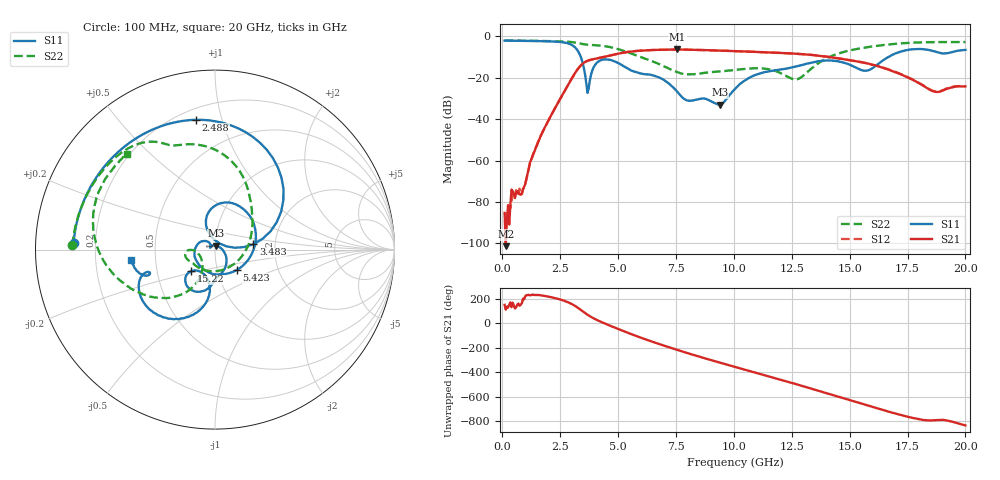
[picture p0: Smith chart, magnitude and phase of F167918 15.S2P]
!  2-Port S-parameters saved by WinCal
! VAR MeasName=S-Parameters (CALIBRATED_DATA) read from VNA (N5242A)
! VAR MeasDate=2016-11-22 10:25:31
! VAR NAME=F167918 15
! VAR FILENAME=F167918 15.S2P
! VAR DATE=2016-11-22 10:25:31
! VAR PHYS_PORTS=1,2
# Hz S DB R 50
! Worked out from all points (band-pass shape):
!   401 points, 100 MHz to 20 GHz, reference 50 ohm
!   highest |S21| = -6.37 dB at 7.562 GHz (marker M1); lowest = -101.4 dB at 149.8 MHz (marker M2)
!   |S21| within 3 dB of the highest: 4.617 GHz to 13.66 GHz (9.042 GHz wide, 98.9 % of centre)
!   lowest |S11| = -33.1 dB at 9.403 GHz (marker M3), VSWR 1.05, Z = 50.7 + j2.14 ohm
!   |S11| at or under -10 dB: 3.391 GHz to 16.67 GHz (13.28 GHz wide, 132 % of centre)
!   |S22| runs from -20.9 to -2.0 dB; largest |S21 - S12| = 0.0044
!   S11 on the Smith chart (normalised r, x): 100 MHz: 0.12, +0.02; 2.488 GHz: 0.27, +0.83; 3.483 GHz: 1.54, +0.10; 5.423 GHz: 1.24, -0.29; 15.22 GHz: 0.74, -0.19; 20 GHz: 0.36, -0.05
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1e8  -2.07 177.3  -85.33 148.6  -85.97 171.1  -2.00 178.3
1.4975e8  -2.07 176.0  -101.39 109.5  -85.49 150.5  -2.01 177.5
8.96e8  -2.18 156.0  -73.81 -160.8  -73.68 177.3  -2.12 165.5
1.44325e9  -2.28 140.1  -53.92 -131.0  -53.94 -129.4  -2.20 156.6
2.488e9  -2.72 98.3  -30.49 -166.7  -30.50 -167.3  -2.43 137.4
3.085e9  -4.78 52.6  -18.76 146.7  -18.78 146.5  -2.91 123.2
3.43325e9  -11.35 12.7  -13.60 101.9  -13.59 101.9  -3.66 115.7
3.483e9  -13.30 8.0  -13.12 95.0  -13.10 94.9  -3.76 115.0
3.682e9  -27.33 51.7  -11.84 68.4  -11.81 68.2  -4.06 112.3
4.279e9  -11.43 78.2  -10.24 9.0  -10.24 8.7  -4.55 99.3
5.42325e9  -15.60 -43.3  -7.56 -78.7  -7.55 -78.7  -7.74 65.5
6.7665e9  -19.84 163.3  -6.50 -169.8  -6.50 -170.0  -13.40 20.3
7.5625e9  -26.89 129.5  -6.37 141.6  -6.40 141.5  -17.35 -33.6
9.40325e9  -33.05 71.2  -6.90 38.2  -6.91 38.2  -16.93 -144.5
1.005e10  -25.37 -15.8  -7.13 3.7  -7.15 3.8  -16.27 -155.2
1.169175e10  -16.57 -82.2  -7.88 -82.9  -7.85 -82.8  -16.46 -178.4
1.268675e10  -14.55 -93.3  -8.39 -136.6  -8.37 -136.5  -20.85 -150.7
1.338325e10  -12.63 -103.7  -9.02 -175.6  -8.97 -175.3  -15.27 -118.7
1.5224e10  -14.87 -137.9  -11.91 82.3  -11.89 82.2  -6.32 -150.0
1.67165e10  -9.72 -102.0  -16.20 -2.1  -16.13 -1.7  -3.91 -177.1
1.865675e10  -7.29 -160.3  -26.65 -70.7  -26.58 -71.0  -2.79 150.3
2e10  -6.56 -173.1  -24.25 -112.9  -24.15 -113.7  -2.77 132.7
